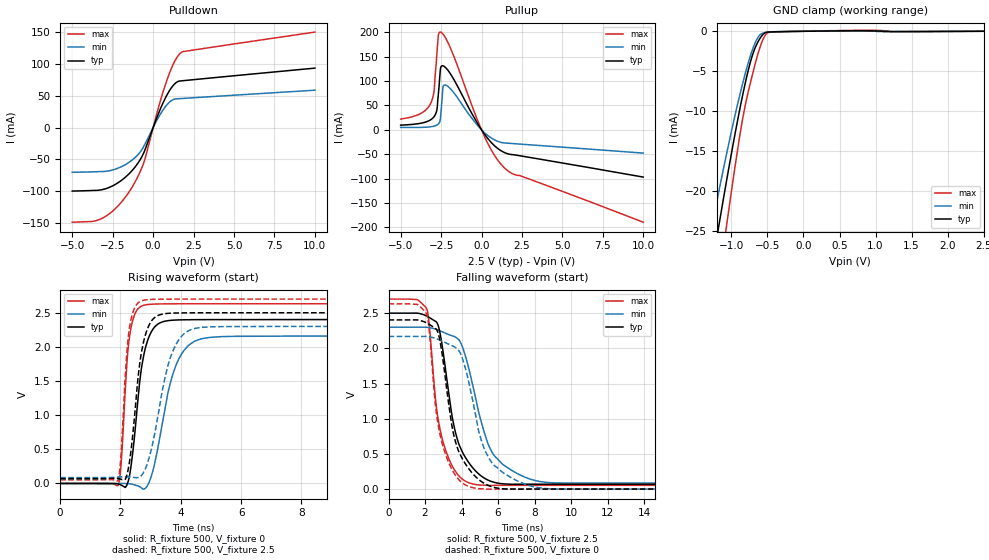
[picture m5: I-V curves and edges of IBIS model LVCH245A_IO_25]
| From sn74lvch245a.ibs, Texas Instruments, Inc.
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[Model]   LVCH245A_IO_25
Model_type  I/O
Vinl=0.7
Vinh=1.7
Enable   Active-Low
Vref =   0
Rref =   500
Cref =   30p
Vmeas =   1.25
| variable   typ   min   max
C_comp   4.44pF   4.13pF   4.98pF
| C_pullup   6.15pF   5.01pF   6.73pF
| C_pulldown   5.44pF   3.66pF   7.50pF
| C_tri-state   4.44pF   4.13pF   4.98pF
[Temperature Range]   40   100   -40
| Ambient temperature   25   85   -40
[Voltage range]   2.5   2.3   2.7
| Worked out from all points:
|   slope of the pulldown table from 0 to 0.375 V, typ, clamps not added: 15 ohm
|   slope of the pullup table from 0 to 0.375 V, typ, clamps not added: 21.7 ohm
|   GND clamp passes 1 mA (typ) near -0.61 V on its own axis
|   rising waveform, R_fixture 500, V_fixture 0: 20-80 % time 378ps typ, 639ps min, 230ps max; typ from 0 V to 2.4 V
|   falling waveform, R_fixture 500, V_fixture 2.5: 20-80 % time 1.04ns typ, 1.41ns min, 804ps max; typ from 2.5 V to 0.069 V
|   rising waveform, R_fixture 500, V_fixture 2.5: 20-80 % time 369ps typ, 628ps min, 224ps max; typ from 0.069 V to 2.5 V
|   falling waveform, R_fixture 500, V_fixture 0: 20-80 % time 1.01ns typ, 1.32ns min, 801ps max; typ from 2.4 V to 0 V
[GND Clamp]
| LVCH245A_IO_25
|   Voltage   I(typ)   I(min)   I(max)
-5V       -263.6mA   -221.9mA   -331mA
-1.27V    -29.57mA   -24.41mA   -38.04mA
-1.19V    -25.22mA   -20.77mA   -32.56mA
-1.15V    -23.08mA   -18.99mA   -29.86mA
-1.075V   -19.15mA   -15.72mA   -24.9mA
-1.04V    -17.36mA   -14.24mA   -22.63mA
-865mV    -8.963mA   -7.319mA   -12.1mA
-750mV    -4.341mA   -3.49mA    -6.98mA
-625mV    -1.231mA   -697.5uA   -2.65mA
-565mV    -445.4uA   -253.1uA   -1.111mA
-505mV    -110.4uA   -130.3uA   -238.5uA
2.5V      21.11pA    82.9nA     -15.29nA
[Pulldown]
| LVCH245A_IO_25
|   Voltage   I(typ)   I(min)   I(max)
-5V       -100.1mA   -70.43mA   -149.1mA
-3.72V    -99.13mA   -69.76mA   -147.8mA
-3.06V    -97.25mA   -69.2mA    -141.7mA
-2.215V   -87.66mA   -64.4mA    -124.6mA
-1.405V   -70.59mA   -53.26mA   -98.19mA
-920mV    -55.28mA   -42.15mA   -75.82mA
-560mV    -38.59mA   -28.63mA   -54.05mA
305mV     20.59mA    15mA       29.32mA
790mV     48.24mA    33.99mA    70.12mA
1.285V    67.66mA    44.56mA    102mA
1.715V    73.53mA    45.7mA     117.9mA
10V       93.67mA    58.88mA    150.5mA
[Pullup]
| LVCH245A_IO_25
|   Voltage   I(typ)   I(min)   I(max)
-5V       9.604mA    4.964mA    22.07mA
-3.76V    13.45mA    4.99mA     33.49mA
-3.13V    20.97mA    6.325mA    55.35mA
-2.93V    27.22mA    7.65mA     81.34mA
-2.76V    41.09mA    9.89mA     155.9mA
-2.665V   74.5mA     12.29mA    194.6mA
-2.51V    129.1mA    34.7mA     200.3mA
-2.385V   131.4mA    87.78mA    196.7mA
-2.18V    126.3mA    91.28mA    186mA
160mV     -7.829mA   -5.242mA   -12.12mA
1.445V    -47.09mA   -27.15mA   -79.1mA
10V       -97.06mA   -47.8mA    -189.7mA
[Ramp]
| LVCH245A_IO_25
| variable   typ   min   max
dV/dt_r   1.48/3.97E-10   1.35/6.70E-10   1.60/2.43E-10
dV/dt_f   1.46/1.06E-09   1.33/1.49E-09   1.59/8.08E-10
R_load = 500
[Rising Waveform]
| LVCH245A_IO_25
R_fixture =   500
C_fixture =   0
L_fixture =   0
V_fixture =   0
V_fixture_min = 0
V_fixture_max = 0
|   Time   V(typ)   V(min)   V(max)
0s        235.2pV    4.368nV    30.83nV
1.92ns    -7.081mV   -1.058mV   -31.27mV
2.015ns   -22.3mV    -436.8uV   248.7mV
2.225ns   -10.23mV   -1.699mV   1.824V
2.335ns   205.5mV    -6.958mV   2.244V
2.675ns   1.618V     -58.51mV   2.591V
2.915ns   2.111V     -16.16mV   2.62V
3.87ns    2.394V     1.761V     2.631V
4.96ns    2.399V     2.139V     2.631V
50ns      2.4V       2.158V     2.631V
[Falling Waveform]
| LVCH245A_IO_25
R_fixture =   500
C_fixture =   0
L_fixture =   0
V_fixture =   2.5
V_fixture_min = 2.3
V_fixture_max = 2.7
|   Time   V(typ)   V(min)   V(max)
0s        2.5V       2.3V       2.7V
2.11ns    2.457V     2.299V     2.548V
2.66ns    2.361V     2.265V     1.095V
3.025ns   1.885V     2.226V     635.7mV
3.675ns   796.8mV    2.158V     247.7mV
4.095ns   501.9mV    1.987V     131.8mV
4.725ns   269.7mV    1.35V      67.5mV
5.81ns    94.34mV    470.3mV    52.74mV
8.635ns   69.05mV    95.21mV    53.29mV
50ns      69.15mV    85.8mV     53.13mV
[Rising Waveform]
| LVCH245A_IO_25
R_fixture =   500
C_fixture =   0
L_fixture =   0
V_fixture =   2.5
V_fixture_min = 2.3
V_fixture_max = 2.7
|   Time   V(typ)   V(min)   V(max)
0s        69.1mV     85.76mV    53.11mV
1.92ns    72.69mV    93.95mV    41.38mV
2.01ns    62.65mV    95.6mV     367.6mV
2.175ns   73.45mV    96.97mV    1.689V
2.295ns   303.8mV    94.95mV    2.268V
2.63ns    1.723V     92.06mV    2.659V
2.865ns   2.228V     259.2mV    2.69V
3.705ns   2.494V     1.901V     2.699V
4.695ns   2.499V     2.285V     2.7V
50ns      2.5V       2.3V       2.7V
[Falling Waveform]
| LVCH245A_IO_25
R_fixture =   500
C_fixture =   0
L_fixture =   0
V_fixture =   0
V_fixture_min = 0
V_fixture_max = 0
|   Time   V(typ)   V(min)   V(max)
0s        2.404V     2.169V     2.632V
2.11ns    2.359V     2.167V     2.475V
2.65ns    2.259V     2.134V     1.027V
3.63ns    709.2mV    2.018V     209.2mV
4.09ns    408.5mV    1.823V     78.28mV
4.725ns   188mV      1.112V     13.77mV
5.155ns   94.94mV    635.7mV    3.257mV
5.74ns    27.29mV    349.3mV    -1.044mV
8.575ns   -69.05uV   7.627mV    169uV
50ns      48.85uV    114.9uV    17.38uV
